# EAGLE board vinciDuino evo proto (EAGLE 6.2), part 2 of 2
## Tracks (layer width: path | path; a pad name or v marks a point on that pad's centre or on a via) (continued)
N$782  (via drill 0.9 pad 1.93)
  other vias: 22.86,83.82
N$783  (via drill 0.9 pad 1.93)
  other vias: 22.86,81.28
N$784  (via drill 0.9 pad 1.93)
  other vias: 22.86,78.74
N$785  (via drill 0.9 pad 1.93)
  other vias: 20.32,78.74
N$786  (via drill 0.9 pad 1.93)
  other vias: 20.32,81.28
N$787  (via drill 0.9 pad 1.93)
  other vias: 20.32,83.82
N$788  (via drill 0.9 pad 1.93)
  other vias: 20.32,86.36
N$789  (via drill 0.9 pad 1.93)
  other vias: 20.32,88.9
N$790  (via drill 0.9 pad 1.93)
  other vias: 20.32,91.44
N$791  (via drill 0.9 pad 1.93)
  other vias: 17.78,91.44
N$792  (via drill 0.9 pad 1.93)
  other vias: 17.78,88.9
N$793  (via drill 0.9 pad 1.93)
  other vias: 17.78,86.36
N$794  (via drill 0.9 pad 1.93)
  other vias: 17.78,83.82
N$795  (via drill 0.9 pad 1.93)
  other vias: 17.78,81.28
N$796  (via drill 0.9 pad 1.93)
  other vias: 17.78,78.74
N$797  (via drill 0.9 pad 1.93)
  other vias: 15.24,78.74
N$798  (via drill 0.9 pad 1.93)
  other vias: 15.24,81.28
N$799  (via drill 0.9 pad 1.93)
  other vias: 15.24,83.82
N$800  (via drill 0.9 pad 1.93)
  other vias: 15.24,86.36
N$801  (via drill 0.9 pad 1.93)
  other vias: 15.24,88.9
N$802  (via drill 0.9 pad 1.93)
  other vias: 15.24,91.44
N$803  (via drill 0.9 pad 1.93)
  other vias: 12.7,91.44
N$804  (via drill 0.9 pad 1.93)
  other vias: 12.7,88.9
N$805  (via drill 0.9 pad 1.93)
  other vias: 12.7,86.36
N$806  (via drill 0.9 pad 1.93)
  other vias: 12.7,83.82
N$807  (via drill 0.9 pad 1.93)
  other vias: 12.7,81.28
N$808  (via drill 0.9 pad 1.93)
  other vias: 12.7,78.74
N$809  (via drill 0.9 pad 1.93)
  other vias: 10.16,78.74
N$810  (via drill 0.9 pad 1.93)
  other vias: 10.16,81.28
N$811  (via drill 0.9 pad 1.93)
  other vias: 10.16,83.82
N$812  (via drill 0.9 pad 1.93)
  other vias: 10.16,86.36
N$813  (via drill 0.9 pad 1.93)
  other vias: 10.16,88.9
N$814  (via drill 0.9 pad 1.93)
  other vias: 10.16,91.44
N$815  (via drill 0.9 pad 1.93)
  other vias: 7.62,78.74
N$816  (via drill 0.9 pad 1.93)
  other vias: 7.62,81.28
N$817  (via drill 0.9 pad 1.93)
  other vias: 7.62,83.82
N$818  (via drill 0.9 pad 1.93)
  other vias: 7.62,86.36
N$819  (via drill 0.9 pad 1.93)
  other vias: 7.62,88.9
N$820  (via drill 0.9 pad 1.93)
  other vias: 7.62,91.44
N$821  (via drill 0.9 pad 1.93)
  other vias: 40.64,93.98
N$822  (via drill 0.9 pad 1.93)
  other vias: 38.1,93.98
N$823  (via drill 0.9 pad 1.93)
  other vias: 35.56,93.98
N$824  (via drill 0.9 pad 1.93)
  other vias: 33.02,93.98
N$825  (via drill 0.9 pad 1.93)
  other vias: 30.48,93.98
N$826  (via drill 0.9 pad 1.93)
  other vias: 27.94,93.98
N$827  (via drill 0.9 pad 1.93)
  other vias: 25.4,93.98
N$828  (via drill 0.9 pad 1.93)
  other vias: 22.86,93.98
N$829  (via drill 0.9 pad 1.93)
  other vias: 20.32,93.98
N$830  (via drill 0.9 pad 1.93)
  other vias: 17.78,93.98
N$831  (via drill 0.9 pad 1.93)
  other vias: 15.24,93.98
N$832  (via drill 0.9 pad 1.93)
  other vias: 12.7,93.98
N$833  (via drill 0.9 pad 1.93)
  other vias: 10.16,93.98
N$834  (via drill 0.9 pad 1.93)
  other vias: 7.62,93.98
N$835  (via drill 0.9 pad 1.93)
  other vias: 86.36,86.36
N$836  (via drill 0.9 pad 1.93)
  other vias: 86.36,83.82
N$837  (via drill 0.9 pad 1.93)
  other vias: 86.36,81.28
N$838  (via drill 0.9 pad 1.93)
  other vias: 88.9,78.74
N$839  (via drill 0.9 pad 1.93)
  other vias: 86.36,93.98
N$840  (via drill 0.35)
  Top 0.406: v91.19,22.1 91.19,21.59 90.55,20.95 89.28,20.95 C7.1
  Top 0.61: C7.1 89.16,17.98 IC1.3
  Bottom 0.406: 3.3V.3 90.17,23.11 v91.19,22.1
N$841  (via drill 0.9 pad 1.93)
  other vias: 86.36,78.74
N$849  (via drill 0.9 pad 1.93)
  other vias: 5.08,73.66
N$850  (via drill 0.9 pad 1.93)
  other vias: 5.08,76.2
N$851  (via drill 0.9 pad 1.93)
  other vias: 5.08,78.74
N$852  (via drill 0.9 pad 1.93)
  other vias: 5.08,81.28
N$853  (via drill 0.9 pad 1.93)
  other vias: 5.08,83.82
N$854  (via drill 0.9 pad 1.93)
  other vias: 5.08,86.36
N$855  (via drill 0.9 pad 1.93)
  other vias: 5.08,88.9
N$856  (via drill 0.9 pad 1.93)
  other vias: 5.08,91.44
N$857  (via drill 0.9 pad 1.93)
  other vias: 83.82,91.44
N$858  (via drill 0.9 pad 1.93)
  other vias: 83.82,88.9
N$859  (via drill 0.9 pad 1.93)
  other vias: 83.82,86.36
N$860  (via drill 0.9 pad 1.93)
  other vias: 83.82,83.82
N$861  (via drill 0.9 pad 1.93)
  other vias: 83.82,81.28
N$862  (via drill 0.9 pad 1.93)
  other vias: 83.82,78.74
N$863  (via drill 0.9 pad 1.93)
  other vias: 81.28,78.74
N$864  (via drill 0.9 pad 1.93)
  other vias: 81.28,81.28
N$865  (via drill 0.9 pad 1.93)
  other vias: 81.28,83.82
N$866  (via drill 0.9 pad 1.93)
  other vias: 81.28,86.36
N$867  (via drill 0.9 pad 1.93)
  other vias: 81.28,88.9
N$868  (via drill 0.9 pad 1.93)
  other vias: 81.28,91.44
N$869  (via drill 0.9 pad 1.93)
  other vias: 78.74,91.44
N$870  (via drill 0.9 pad 1.93)
  other vias: 78.74,88.9
N$871  (via drill 0.9 pad 1.93)
  other vias: 78.74,86.36
N$872  (via drill 0.9 pad 1.93)
  other vias: 78.74,83.82
N$873  (via drill 0.9 pad 1.93)
  other vias: 78.74,81.28
N$874  (via drill 0.9 pad 1.93)
  other vias: 78.74,78.74
N$875  (via drill 0.9 pad 1.93)
  other vias: 76.2,78.74
N$876  (via drill 0.9 pad 1.93)
  other vias: 76.2,81.28
N$877  (via drill 0.9 pad 1.93)
  other vias: 76.2,83.82
N$878  (via drill 0.9 pad 1.93)
  other vias: 76.2,86.36
N$879  (via drill 0.9 pad 1.93)
  other vias: 76.2,88.9
N$880  (via drill 0.9 pad 1.93)
  other vias: 76.2,91.44
N$881  (via drill 0.9 pad 1.93)
  other vias: 73.66,91.44
N$882  (via drill 0.9 pad 1.93)
  other vias: 73.66,88.9
N$883  (via drill 0.9 pad 1.93)
  other vias: 73.66,86.36
N$884  (via drill 0.9 pad 1.93)
  other vias: 73.66,83.82
N$885  (via drill 0.9 pad 1.93)
  other vias: 73.66,81.28
N$886  (via drill 0.9 pad 1.93)
  other vias: 73.66,78.74
N$887  (via drill 0.9 pad 1.93)
  other vias: 71.12,78.74
N$888  (via drill 0.9 pad 1.93)
  other vias: 71.12,81.28
N$889  (via drill 0.9 pad 1.93)
  other vias: 71.12,83.82
N$890  (via drill 0.9 pad 1.93)
  other vias: 71.12,86.36
N$891  (via drill 0.9 pad 1.93)
  other vias: 71.12,88.9
N$892  (via drill 0.9 pad 1.93)
  other vias: 71.12,91.44
N$893  (via drill 0.9 pad 1.93)
  other vias: 68.58,91.44
N$894  (via drill 0.9 pad 1.93)
  other vias: 68.58,88.9
N$895  (via drill 0.9 pad 1.93)
  other vias: 68.58,86.36
N$896  (via drill 0.9 pad 1.93)
  other vias: 68.58,83.82
N$897  (via drill 0.9 pad 1.93)
  other vias: 68.58,81.28
N$898  (via drill 0.9 pad 1.93)
  other vias: 68.58,78.74
N$899  (via drill 0.9 pad 1.93)
  other vias: 66.04,78.74
N$900  (via drill 0.9 pad 1.93)
  other vias: 66.04,81.28
N$901  (via drill 0.9 pad 1.93)
  other vias: 66.04,83.82
N$902  (via drill 0.9 pad 1.93)
  other vias: 66.04,86.36
N$903  (via drill 0.9 pad 1.93)
  other vias: 66.04,88.9
N$904  (via drill 0.9 pad 1.93)
  other vias: 66.04,91.44
N$905  (via drill 0.9 pad 1.93)
  other vias: 63.5,91.44
N$906  (via drill 0.9 pad 1.93)
  other vias: 63.5,88.9
N$907  (via drill 0.9 pad 1.93)
  other vias: 63.5,86.36
N$908  (via drill 0.9 pad 1.93)
  other vias: 63.5,83.82
N$909  (via drill 0.9 pad 1.93)
  other vias: 63.5,81.28
N$910  (via drill 0.9 pad 1.93)
  other vias: 63.5,78.74
N$911  (via drill 0.9 pad 1.93)
  other vias: 60.96,78.74
N$912  (via drill 0.9 pad 1.93)
  other vias: 60.96,81.28
N$913  (via drill 0.9 pad 1.93)
  other vias: 60.96,83.82
N$914  (via drill 0.9 pad 1.93)
  other vias: 60.96,86.36
N$915  (via drill 0.9 pad 1.93)
  other vias: 60.96,88.9
N$916  (via drill 0.9 pad 1.93)
  other vias: 60.96,91.44
N$917  (via drill 0.9 pad 1.93)
  other vias: 58.42,91.44
N$918  (via drill 0.9 pad 1.93)
  other vias: 58.42,88.9
N$919  (via drill 0.9 pad 1.93)
  other vias: 58.42,86.36
N$920  (via drill 0.9 pad 1.93)
  other vias: 58.42,83.82
N$921  (via drill 0.9 pad 1.93)
  other vias: 58.42,81.28
N$922  (via drill 0.9 pad 1.93)
  other vias: 58.42,78.74
N$923  (via drill 0.9 pad 1.93)
  other vias: 55.88,78.74
N$924  (via drill 0.9 pad 1.93)
  other vias: 55.88,81.28
N$925  (via drill 0.9 pad 1.93)
  other vias: 55.88,83.82
N$926  (via drill 0.9 pad 1.93)
  other vias: 55.88,86.36
N$927  (via drill 0.9 pad 1.93)
  other vias: 55.88,88.9
N$928  (via drill 0.9 pad 1.93)
  other vias: 55.88,91.44
N$929  (via drill 0.9 pad 1.93)
  other vias: 53.34,91.44
N$930  (via drill 0.9 pad 1.93)
  other vias: 53.34,88.9
N$931  (via drill 0.9 pad 1.93)
  other vias: 53.34,86.36
N$932  (via drill 0.9 pad 1.93)
  other vias: 53.34,83.82
N$933  (via drill 0.9 pad 1.93)
  other vias: 53.34,81.28
N$934  (via drill 0.9 pad 1.93)
  other vias: 53.34,78.74
N$935  (via drill 0.9 pad 1.93)
  other vias: 50.8,78.74
N$936  (via drill 0.9 pad 1.93)
  other vias: 50.8,81.28
N$937  (via drill 0.9 pad 1.93)
  other vias: 50.8,83.82
N$938  (via drill 0.9 pad 1.93)
  other vias: 50.8,86.36
N$939  (via drill 0.9 pad 1.93)
  other vias: 50.8,88.9
N$940  (via drill 0.9 pad 1.93)
  other vias: 50.8,91.44
N$941  (via drill 0.9 pad 1.93)
  other vias: 48.26,91.44
N$942  (via drill 0.9 pad 1.93)
  other vias: 48.26,88.9
N$943  (via drill 0.9 pad 1.93)
  other vias: 48.26,86.36
N$944  (via drill 0.9 pad 1.93)
  other vias: 48.26,83.82
N$945  (via drill 0.9 pad 1.93)
  other vias: 48.26,81.28
N$946  (via drill 0.9 pad 1.93)
  other vias: 48.26,78.74
N$948  (via drill 0.9 pad 1.93)
  other vias: 83.82,93.98
N$949  (via drill 0.9 pad 1.93)
  other vias: 81.28,93.98
N$952  (via drill 0.9 pad 1.93)
  other vias: 78.74,93.98
N$953  (via drill 0.9 pad 1.93)
  other vias: 76.2,93.98
N$956  (via drill 0.9 pad 1.93)
  other vias: 73.66,93.98
N$957  (via drill 0.9 pad 1.93)
  other vias: 71.12,93.98
N$960  (via drill 0.9 pad 1.93)
  other vias: 68.58,93.98
N$961  (via drill 0.9 pad 1.93)
  other vias: 66.04,93.98
N$964  (via drill 0.9 pad 1.93)
  other vias: 63.5,93.98
N$965  (via drill 0.9 pad 1.93)
  other vias: 60.96,93.98
N$968  (via drill 0.9 pad 1.93)
  other vias: 58.42,93.98
N$969  (via drill 0.9 pad 1.93)
  other vias: 55.88,93.98
N$972  (via drill 0.9 pad 1.93)
  other vias: 53.34,93.98
N$973  (via drill 0.9 pad 1.93)
  other vias: 50.8,93.98
N$976  (via drill 0.9 pad 1.93)
  other vias: 48.26,93.98
N$977  (via drill 0.9 pad 1.93)
  other vias: 45.72,78.74
N$978  (via drill 0.9 pad 1.93)
  other vias: 45.72,81.28
N$979  (via drill 0.9 pad 1.93)
  other vias: 45.72,83.82
N$980  (via drill 0.9 pad 1.93)
  other vias: 45.72,86.36
N$981  (via drill 0.9 pad 1.93)
  other vias: 45.72,88.9
N$982  (via drill 0.9 pad 1.93)
  other vias: 45.72,91.44
N$983  (via drill 0.9 pad 1.93)
  other vias: 43.18,91.44
N$984  (via drill 0.9 pad 1.93)
  other vias: 43.18,88.9
N$985  (via drill 0.9 pad 1.93)
  other vias: 43.18,86.36
N$986  (via drill 0.9 pad 1.93)
  other vias: 43.18,83.82
N$987  (via drill 0.9 pad 1.93)
  other vias: 43.18,81.28
N$988  (via drill 0.9 pad 1.68)
  other vias: 43.18,78.74
N$989  (via drill 0.9 pad 1.93)
  other vias: 45.72,93.98
N$990  (via drill 0.9 pad 1.93)
  other vias: 43.18,93.98
N$993  (via drill 0.9 pad 1.93)
  other vias: 88.9,91.44
N$994  (via drill 0.9 pad 1.93)
  other vias: 88.9,88.9
N$995  (via drill 0.9 pad 1.93)
  other vias: 88.9,86.36
N$996  (via drill 0.9 pad 1.93)
  other vias: 88.9,83.82
N$997  (via drill 0.9 pad 1.93)
  other vias: 88.9,81.28
N$1000  (via drill 0.9 pad 1.93)
  other vias: 88.9,93.98
RESET  (via drill 0.35)
  Top 0.305: U1.13 65.38,36.22 64.77,36.83 64.77,45.09 v65.53,45.85 | JP3.5 76.32,48.26 C2.2 | S2.3 | 85.09,48.13 87.38,48.13 v88.27,47.24 | S2.4 84.58,48.01
  Top 0.406: S2.4 S2.3 | S2.3 C2.2 | R2.1 84.19,46.35 84.58,46.74 84.58,48.01 84.84,48.01 | 84.84,48.01 85.09,48.26 | 84.84,48.01 84.96,48.01 85.09,48.13
  Bottom 0.305: v65.53,45.85 66.17,45.21 72.52,45.21 73.66,46.35 JP3.5
  Bottom 0.406: v88.27,47.24 88.52,46.99 88.52,23.24 93.98,17.78 JP4.3
RST
  Bottom 0.305: JP2.1 71.5,0.89 87.12,0.89 87.63,1.4 AUTO-RESET.1
RX-I  (via drill 0.9 pad 1.68)
  Top 0.305: U1.20 56.38,30.62 53.98,33.02 53.98,46.35 52.07,48.26 J1.1
  Top 0.406: J1.1 v43.18,48.26
  Bottom 0.305: JP2.3 74.93,11.3 86.87,23.24 86.87,42.04 84.58,44.2 63.75,44.2 59.69,48.26 J1.1
RXLED  (via drill 0.35)
  Top 0.254: v72.14,21.59 72.39,21.34 73.41,21.34 74.04,20.7 R7.1
  Top 0.305: U1.8 70.79,40.34 v70.74,40.26
  Bottom 0.305: v70.74,40.26 70.74,35.81 72.26,34.29 v72.14,21.59
SCK
  Top 0.305: U1.9 69.99,46.65 71.12,47.78 JP3.3
TX-O  (via drill 0.9 pad 1.68)
  Top 0.305: U1.21 55.91,29.82 53.21,32.51 53.21,44.58 52.07,45.72 J1.2
  Top 0.406: J1.2 v43.18,45.72
  Bottom 0.305: JP2.2 72.39,10.79 85.85,24.26 85.85,40.89 83.57,43.18 62.23,43.18 59.69,45.72 J1.2
TXLED  (via drill 0.35)
  Top 0.254: R8.1 71.5,20.57 v71.37,20.7
  Top 0.305: v60.45,26.8 60.45,27.81 61.66,29.02 U1.22
  Bottom 0.305: v60.45,26.8 60.45,22.99 61.85,21.59 70.48,21.59 v71.37,20.7
VCC  (via drill 0.35, 0.9 pad 1.68, 0.9 pad 1.93)
  Top 0.203: v43.18,58.42 44.45,57.15 87.63,57.15 v88.9,58.42
  Top 0.254: 65.15,35.43 65.08,35.43
  Top 0.305: 75.59,35.56 75.59,30.33 76.9,29.02 U1.34 78.13,28.96 | 75.59,35.56 U1.2 75.59,40.41 79.63,44.45 R2.2 | 66.6,35.43 U1.14 66.58,35.43 | 75.18,35.43 75.46,35.43 75.59,35.56 | 75.18,35.43 72.01,35.43 | 72.01,35.43 71.75,35.43 | 71.75,35.43 71.25,35.43 | 71.75,35.43 71.59,35.6 U1.7 71.59,40.68 70.99,41.27 70.99,43.95 C4.1 71.5,46.23 v70.83,46.23 | 71.25,35.43 71.63,35.81 72.01,35.43 | 75.18,35.43 75.56,35.81 | 75.18,35.43 75.56,35.05 | 77.6,17.78 69.34,17.78 68.96,18.16 68.58,19.05 | 71.25,35.43 69.98,35.43 v68.07,33.53 | v59.82,43.31 C9.1
  Top 0.406: 68.56,19.2 R11.2 68.48,19.3 | 78.13,28.96 78.13,25.63 79.12,24.64 C10.1 | C10.1 | C10.1 83.77,24.64 L1.1 | 66.58,35.43 65.15,35.43 | C9.1 62.04,42.61 63.88,40.77 63.88,36.64 65.08,35.43 | 74.17,9.78 74.04,9.78 RX.A | 77.6,17.78 77.72,17.78 80.64,20.7 | 80.64,20.7 | C8.A 80.64,20.7 | JP4.5 98.04,21.34 98.04,16.76 JP4.2 | D1.C 65.15,20.83 66.67,19.3 68.33,19.3 68.45,19.18 68.58,19.18
  Top 0.508: C8.A 80.64,19.17 79.5,18.03 79.5,9.02 77.47,6.99 JP2.4
  Top 0.61: L1.1 83.72,24.59 83.72,24.48 83.95,24.26 84.39,24.7 C12.1 C11.1 92.14,24.7 93.98,22.86 JP4.5 | RX.A TX.A | 68.56,19.2 68.56,19.02 | 68.58,19.05 68.58,19.18 R11.2 | C10.1 80.77,20.83 80.64,20.7 | 74.04,9.78 74.04,5.97 JP2.4 81.79,6.86 87.76,6.86 89.15,8.26 C17.2 | 89.28,10.28 C17.2 | IC1.1 89.2,10.46 C17.2
  Bottom 0.305: v70.83,46.23 67.44,46.23 66.83,46.83 66.83,49.05 JP3.2 | v68.07,33.53 64.01,33.53 59.18,38.35 59.18,42.55 v59.82,43.31 | JP4.5 91.69,27.69 91.69,56.9 90.17,58.42 v88.9,58.42

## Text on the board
tPlace: GND | A5 | A5 | A4 | A4 | A3 | A3 | A2 | A2 | A1 | A1 | GND | A0 | A0 | GND | 5V | 5V | 3.3V | 3.3V | GND | 0 | 0 | RX | A5 | ICSP | 1 | Reset | 1 | 1 | TX | A4 | 2 | 2 | A3 | 3 | ~3 | A2 | 4 | 4 | ~ | PWM: | A1 | ANALOG IN | 5 | ~5 | A0 | 6 | ~6 | 7 | 7 | GND | GND | 8 | 8 | GND | DIGITAL | 9 | ~9 | POWER | 5V | 10 | ~10 | 3.3V | 11 | ~11 | RST | 12 | 12 | IOREF | 13 | 13 | GND | GND | ARF | ARF | SDA | SDA | RST | TX | RX | 5V | GND | UART | GND | SCL | SCL
bPlace: Authors and contributors | vinciDuino Team | fmalpartida, Inizul, JMN | nayma, flico, yOPERO | shaktale, GabyCR, josemanu | chiva, Igor R, Terraguea45
bNames: PF0 | PF1 | PF4 | PF5 | PF6 | PF7 | PD2 | PD3 | PD1 | PD0 | PD4 | A6 | PC6 | PD7 | A7 | PE6 | Ain0 | AVR | PB4 | A8 | LDO | PB5 | A9 | PB6 | A10 | PB7 | PD6 | A11 | PC7 | GND | ARF | PD2 | PD3
tDocu: vinciDuino evo Proto | http://creativecommons.org/licenses/by-sa/3.0 | Released under the Creative Commons Attribution Share-Alike 3.0 License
